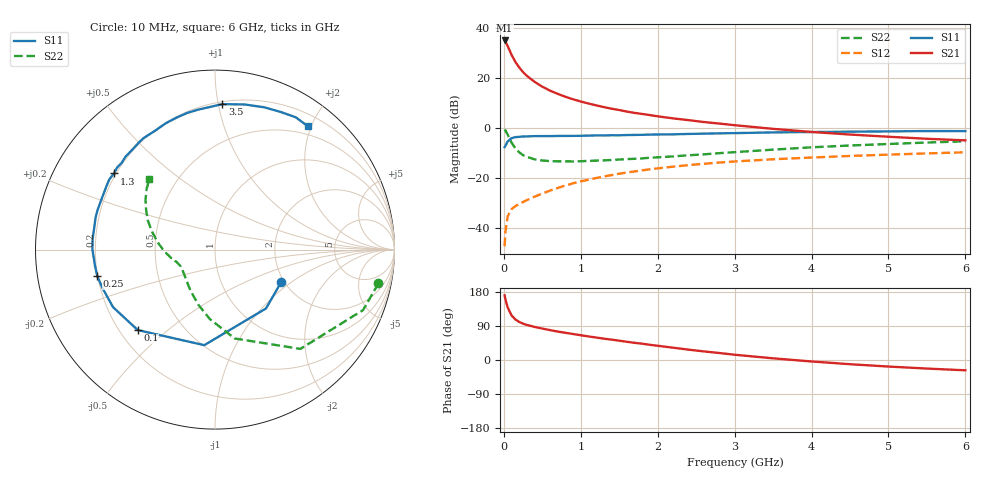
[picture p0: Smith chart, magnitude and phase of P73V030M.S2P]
! SIEMENS Small Signal Semiconductors
! BFP196
! Si NPN RF Bipolar Junction Transistor in SOT143
! VCE = 3 V  IC = 30 mA
! Common Emitter S-Parameters:  May  1996
# GHz  S  MA  R  50
!  f  S11  S21  S12  S22
! GHz  MAG  ANG  MAG  ANG  MAG  ANG  MAG  ANG
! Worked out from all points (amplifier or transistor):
!   36 points, 10 MHz to 6 GHz, reference 50 ohm
!   highest |S21| = 35.0 dB at 10 MHz (marker M1)
!   |S21| within 3 dB of that: start of sweep to 61.03 MHz
!   unconditionally stable (mu >= 1): 544.1 MHz to 4.091 GHz
!   at 250 MHz: K = 0.72, MSG = 26.0 dB, |S12| = -29.7 dB
!   at 1.4 GHz: K = 1.10, MAG = 11.4 dB, |S12| = -18.9 dB
!   at 6 GHz: K = 0.98, MSG = 2.4 dB, |S12| = -9.8 dB
!   lowest NFmin = 1.40 dB at 500 MHz
!   S11 on the Smith chart (normalised r, x): 10 MHz: 1.92, -0.84; 100 MHz: 0.27, -0.40; 250 MHz: 0.20, -0.11; 1.3 GHz: 0.19, +0.32; 3.5 GHz: 0.22, +1.03; 6 GHz: 0.37, +1.95
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0.01  0.4106 -26.4  56.02 170.5  0.0043 79.7  0.9299 -11.7
0.02  0.4339 -49.1  53.02 160.5  0.0082 72.2  0.8912 -22.2
0.05  0.5358 -96.4  43.34 138.6  0.017 57.5  0.7297 -49.3
0.1  0.6214 -133.8  28.99 117.8  0.0237 47.3  0.5073 -77.5
0.15  0.6522 -150.5  20.84 107.0  0.0272 44.9  0.3883 -94.2
0.2  0.6615 -160.6  16.16 100.4  0.0301 44.9  0.3243 -106.0
0.25  0.6724 -167.2  13.02 95.9  0.0329 46.6  0.2841 -115.2
0.3  0.6746 -172.2  10.96 92.6  0.0359 49.7  0.2626 -121.9
0.4  0.6832 179.8  8.324 87.3  0.0421 52.4  0.2349 -132.5
0.5  0.6844 175.0  6.66 83.0  0.0485 54.7  0.2222 -139.8
0.6  0.6837 169.8  5.565 78.9  0.0555 56.5  0.2164 -144.9
0.7  0.6889 165.1  4.791 75.0  0.0626 57.2  0.2141 -148.6
0.9  0.6912 157.3  3.728 68.6  0.0777 57.6  0.2132 -154.5
1.1  0.6997 150.1  3.07 62.2  0.092 56.7  0.2182 -158.4
1.3  0.7049 143.0  2.601 56.3  0.1067 55.2  0.2237 -161.8
1.7  0.7215 130.4  1.992 45.3  0.1344 51.1  0.2405 -167.8
2.2  0.7415 116.8  1.547 32.5  0.1675 44.7  0.2686 -174.7
2.8  0.7768 101.5  1.219 18.5  0.2024 36.7  0.3118 174.8
3.5  0.8115 87.1  0.955 4.4  0.2353 27.3  0.3668 163.7
4.5  0.8391 70.9  0.735 -11.1  0.2743 15.6  0.4437 149.9
5.5  0.8636 58.6  0.605 -22.6  0.3086 4.9  0.5089 138.5
6  0.8602 53.1  0.562 -27.2  0.3246 -0.9  0.5381 132.8
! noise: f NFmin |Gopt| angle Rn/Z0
0.5  1.4  0.4  -173  0.08
0.9  1.6  0.5  -166  0.08
1.5  2.4  0.61  -150  0.14
2  2.9  0.71  -129  0.2
